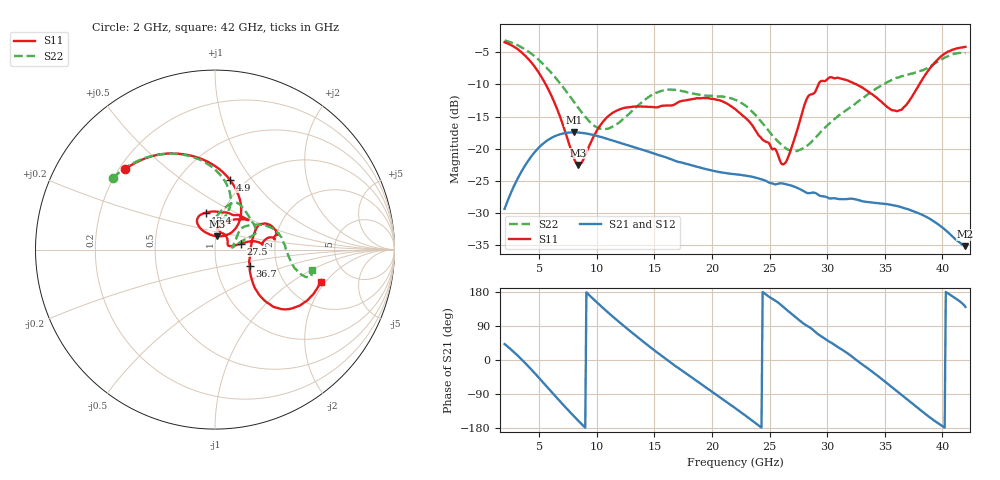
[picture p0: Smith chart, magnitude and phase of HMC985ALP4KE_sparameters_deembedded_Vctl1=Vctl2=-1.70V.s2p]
!s2p File: Measurements: S11, S21, S12, S22
# GHz S dB R 50.0
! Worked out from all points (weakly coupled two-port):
!   401 points, 2 GHz to 42 GHz, reference 50 ohm
!   highest |S21| = -17.44 dB at 8 GHz (marker M1); lowest = -35.1 dB at 42 GHz (marker M2)
!   lowest |S11| = -22.5 dB at 8.4 GHz (marker M3), VSWR 1.16, Z = 50.5 + j7.55 ohm
!   |S11| at or under -10 dB: 5.569 GHz to 29.25 GHz (23.68 GHz wide, 136 % of centre); 32.55 GHz to 38 GHz (5.448 GHz wide, 15.4 % of centre)
!   |S22| runs from -20.4 to -3.2 dB; largest |S21 - S12| = 0.00014
!   S11 on the Smith chart (normalised r, x): 2 GHz: 0.22, +0.36; 4.9 GHz: 0.85, +0.78; 13.4 GHz: 0.83, +0.36; 27.5 GHz: 1.34, +0.09; 36.7 GHz: 1.45, -0.27; 42 GHz: 3.10, -1.81
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2  -3.44 138.4  -29.31 42.0  -29.33 42.1  -3.17 145.0
3.4  -4.92 110.1  -23.73 3.8  -23.74 3.8  -4.17 121.6
4.9  -7.99 78.1  -19.93 -44.3  -19.94 -44.3  -6.08 97.8
6.2  -12.30 53.5  -18.17 -88.6  -18.18 -88.6  -8.49 80.6
8  -21.39 61.9  -17.44 -147.8  -17.45 -147.8  -12.65 70.7
8.4  -22.49 81.8  -17.47 -160.3  -17.47 -160.3  -13.64 71.7
8.7  -22.11 97.2  -17.52 -169.5  -17.52 -169.5  -14.36 73.3
10.7  -15.46 124.4  -18.33 133.0  -18.34 133.0  -16.95 91.5
13.4  -13.43 104.1  -19.83 63.8  -19.84 63.8  -13.55 82.6
15.4  -13.48 78.0  -20.98 16.3  -20.98 16.3  -11.12 69.2
18.9  -12.16 42.5  -22.89 -59.9  -22.89 -59.9  -11.60 43.4
22  -13.81 55.7  -23.94 -126.6  -23.95 -126.6  -12.37 21.5
24.5  -18.71 83.9  -24.84 177.0  -24.85 177.0  -16.25 17.1
26.2  -22.41 19.3  -25.40 139.8  -25.41 139.8  -19.64 8.3
27.5  -16.49 12.9  -26.14 106.8  -26.14 106.7  -20.24 8.2
28.7  -11.51 6.2  -26.80 81.3  -26.81 81.3  -18.80 19.5
31.1  -9.06 18.3  -27.81 30.9  -27.82 31.0  -14.70 38.5
33.3  -10.78 29.1  -28.21 -17.2  -28.21 -17.1  -11.87 32.8
35.4  -13.72 8.9  -28.65 -66.2  -28.65 -66.2  -9.52 21.4
36.7  -13.46 -24.7  -29.22 -98.1  -29.22 -98.1  -8.63 12.3
39.6  -6.13 -42.1  -31.67 -166.3  -31.66 -166.4  -6.48 -14.7
42  -4.16 -16.9  -35.11 140.0  -35.15 140.0  -5.14 -12.0
